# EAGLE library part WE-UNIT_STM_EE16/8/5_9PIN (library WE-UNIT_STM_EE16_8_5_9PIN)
Off-Line Transformer WE-Unit STM - Nominal input voltage: 85-265 VAC - Operating temperature: -40°C to +125 °C - Isolation voltage 4 kVAC -- Especially designed for several ICs from STMicroelectronics VIPer 17L and VIPer 15L -- Universal input -- Offline-switch mode power supplies
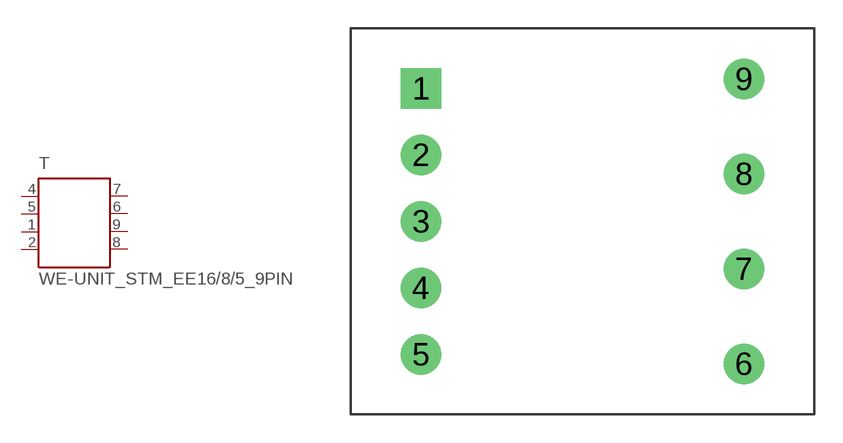
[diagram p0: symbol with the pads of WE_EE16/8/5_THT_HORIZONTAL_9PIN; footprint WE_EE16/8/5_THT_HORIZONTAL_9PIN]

Designator prefix T

## WE-UNIT_STM_EE16/8/5_9PIN-750370026 (MPN: 750370026; OC_FARNELL: 1849047; OC_NEWARK: 13T9836; PACKAGE: EE16/8/5_THT_HORIZONTAL_9PIN; SUPPLIER: Würth Elektronik eiSos GmbH), WE-UNIT_STM_EE16/8/5_9PIN-750871010 (MPN: 750871010; OC_FARNELL: 1849044; OC_NEWARK: 13T9838; PACKAGE: EE16/8/5_THT_HORIZONTAL_9PIN; SUPPLIER: Würth Elektronik eiSos GmbH), WE-UNIT_STM_EE16/8/5_9PIN-750871011 (MPN: 750871011; OC_FARNELL: 1849046; OC_NEWARK: 13T9839; PACKAGE: EE16/8/5_THT_HORIZONTAL_9PIN; SUPPLIER: Würth Elektronik eiSos GmbH), WE-UNIT_STM_EE16/8/5_9PIN-750871030 (MPN: 750871030; OC_FARNELL: 1849045; OC_NEWARK: 13T9841; PACKAGE: EE16/8/5_THT_HORIZONTAL_9PIN; SUPPLIER: Würth Elektronik eiSos GmbH)  [WE_EE16/8/5_THT_HORIZONTAL_9PIN]
1  2  pas
2  1  pas
4  4  pas
5  3  pas
6  6  pas
7  5  pas
8  8  pas
9  7  pas

## Footprint WE_EE16/8/5_THT_HORIZONTAL_9PIN (pad centres in mm)
Transformer, EE16/8/5 THT Horizontal 9 Pin
drill 1.42 square: 1 -8.5,7
drill 1.42: 2 -8.5,3.5; 3 -8.5,0; 4 -8.5,-3.5; 5 -8.5,-7; 6 8.5,-7.5; 7 8.5,-2.5; 8 8.5,2.5; 9 8.5,7.5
